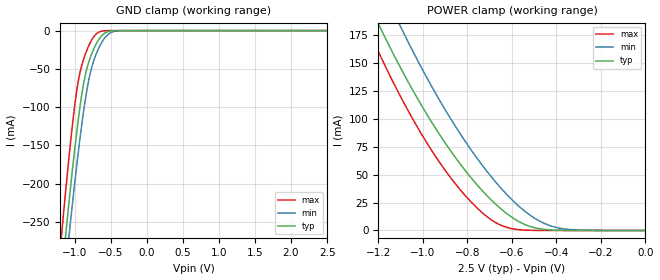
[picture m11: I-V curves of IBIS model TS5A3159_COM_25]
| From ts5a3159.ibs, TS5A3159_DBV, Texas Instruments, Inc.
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[Model]   TS5A3159_COM_25
Model_type  Terminator
| variable   typ   min   max
C_comp   47.98pF   39.11pF   54.07pF
| C_tri-state   47.98pF   39.11pF   54.07pF
[Temperature Range]   40   100   -40
| Ambient temperature   25   85   -40
[Voltage range]   2.5   2.3   2.7
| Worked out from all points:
|   GND clamp passes 1 mA (typ) near -0.52 V on its own axis
|   POWER clamp passes 1 mA (typ) near -0.46 V on its own axis
[GND Clamp]
| TS5A3159_COM_25
|   Voltage   I(typ)   I(min)   I(max)
-2.5V     -1.87A     -1.846A    -1.924A
-1.18V    -321.7mA   -363.4mA   -266.3mA
-1.12V    -263.9mA   -307.1mA   -206.1mA
-1.07V    -217.7mA   -261.7mA   -158.8mA
-990mV    -148.7mA   -192.6mA   -92.1mA
-935mV    -106.6mA   -148.6mA   -59.22mA
-870mV    -66.95mA   -102.2mA   -36.16mA
-805mV    -41.68mA   -65.44mA   -20.03mA
-670mV    -12.38mA   -23.82mA   -2.425mA
-555mV    -1.971mA   -6.693mA   -97.21uA
-415mV    -62.78uA   -521.2uA   -506.6nA
2.5V      3.408nA    33.78uA    2.672nA
[POWER Clamp]
| TS5A3159_COM_25
|   Voltage   I(typ)   I(min)   I(max)
-2.5V     970.9mA    1.037A     1.006A
-1.25V    206.1mA    247.4mA    181.9mA
-1.18V    176.7mA    216mA      151.5mA
-1.105V   147.3mA    184.2mA    121.5mA
-1.085V   139.8mA    176.1mA    114mA
-945mV    91.98mA    123.4mA    66.81mA
-790mV    48.71mA    73.98mA    26.9mA
-675mV    23.88mA    43.76mA    7.285mA
-545mV    5.59mA     17.68mA    357.8uA
-475mV    1.513mA    8.318mA    37.06uA
-385mV    174uA      2.024mA    1.245uA
0V        0A         0A         0A
